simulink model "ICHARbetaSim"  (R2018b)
settings: Solver=ode5  StartTime=0.0  StopTime=80  FixedStep=0.001  RelTol=1e-3  AbsTol=1e-6
libraries: simulink x1

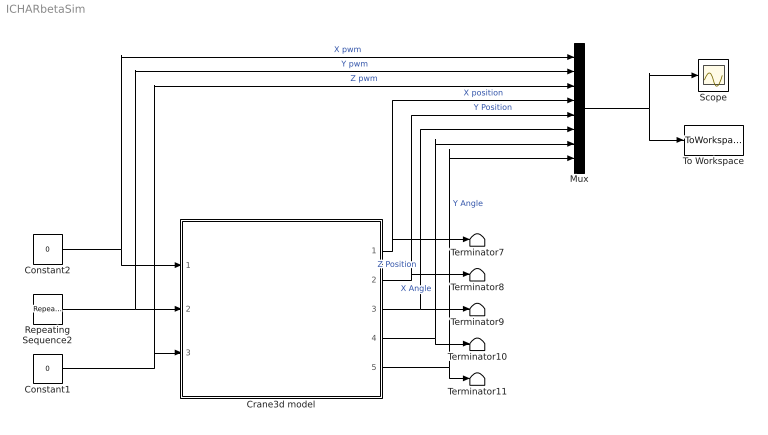
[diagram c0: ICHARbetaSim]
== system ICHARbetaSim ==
  Constant1 : Constant  Value=0
  Constant2 : Constant  Value=0
  Crane3d model : Subsystem  mask{RR=off, x0=[ 0, 0, 0,  0, 0, 0, 0, 0,  0.552, 0, -1]}
      mask prompts: RR "Model with constant length"; x0 "Initial conditions:[x,x',y,y',alfa,alfa',beta,beta',z,z',t]"
  Mux : Mux  Inputs=8
  Repeating Sequence2 : simulink/Sources/Repeating Sequence  rep_seq_t=[0 1.99 2 2.99 3 80]  rep_seq_y=[0 0 1 1 0 0]
  Scope : Scope
  Terminator{7..11} (5 alike) : Terminator
  To Workspace : ToWorkspace  VariableName=ICHARbeta  SaveFormat=Timeseries  SampleTime=-1
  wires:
  Repeating Sequence2/1 -> Crane3d model/2(Y PWM), Mux/2  "Y pwm"
  Constant1/1 -> Crane3d model/3(Z PWM), Mux/3  "Z pwm"
  Constant2/1 -> Crane3d model/1(X PWM), Mux/1  "X pwm"
  Mux/1 -> Scope/1, To Workspace/1
  Crane3d model/1(X Posiion) -> Mux/4, Terminator7/1  "X position"
  Crane3d model/2(Y Position) -> Mux/5, Terminator8/1  "Y Position"
  Crane3d model/5(Y Angle) -> Mux/8, Terminator11/1  "Y Angle"
  Crane3d model/4(X Angle) -> Mux/7, Terminator10/1  "X Angle"
  Crane3d model/3(Z Position) -> Mux/6, Terminator9/1  "Z Position"

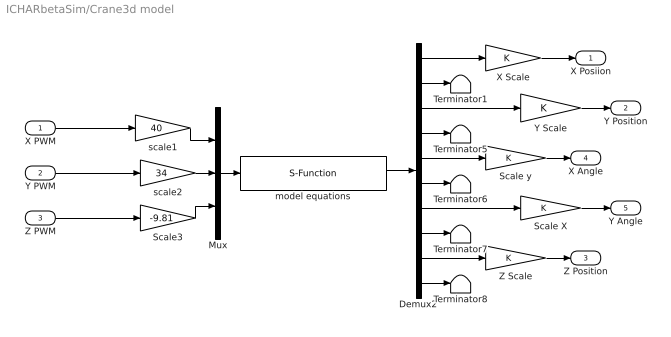
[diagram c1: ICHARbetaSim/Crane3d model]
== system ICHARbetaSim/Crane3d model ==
  X PWM : Inport
  Y PWM : Inport  Port=2
  Z PWM : Inport  Port=3
  Demux2 : Demux  Outputs=10
  Mux : Mux  Inputs=3
  Scale X : Gain
  Scale y : Gain
  Scale3 : Gain  Gain=-9.81
  Terminator{1,5..8} (5 alike) : Terminator
  X Scale : Gain
  Y Scale : Gain
  Z Scale : Gain
  model equations : S-Function  FunctionName=model3dddm  Parameters=x0(1) x0(2) x0(3) x0(4) x0(5) x0(6) x0(7) x0(8) x0(9) x0(10) x0(11) RR  SFunctionDeploymentMode=off  EnableBusSupport=off
  scale1 : Gain  Gain=40
  scale2 : Gain  Gain=34
  X Posiion : Outport  Tag=X Position
  Y Position : Outport  Port=2
  Z Position : Outport  Port=3
  X Angle : Outport  Port=4
  Y Angle : Outport  Port=5
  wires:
  X PWM/1 -> scale1/1
  scale1/1 -> Mux/1
  Z PWM/1 -> Scale3/1
  Scale3/1 -> Mux/3
  Y PWM/1 -> scale2/1
  scale2/1 -> Mux/2
  Demux2/10 -> Terminator8/1
  Demux2/8 -> Terminator7/1
  Demux2/6 -> Terminator6/1
  Demux2/4 -> Terminator5/1
  Demux2/2 -> Terminator1/1
  Demux2/7 -> Scale X/1
  Scale X/1 -> Y Angle/1
  Demux2/5 -> Scale y/1
  Scale y/1 -> X Angle/1
  Demux2/9 -> Z Scale/1
  Z Scale/1 -> Z Position/1
  Demux2/3 -> Y Scale/1
  Demux2/1 -> X Scale/1
  X Scale/1 -> X Posiion/1
  model equations/1 -> Demux2/1
  Y Scale/1 -> Y Position/1
  Mux/1 -> model equations/1
